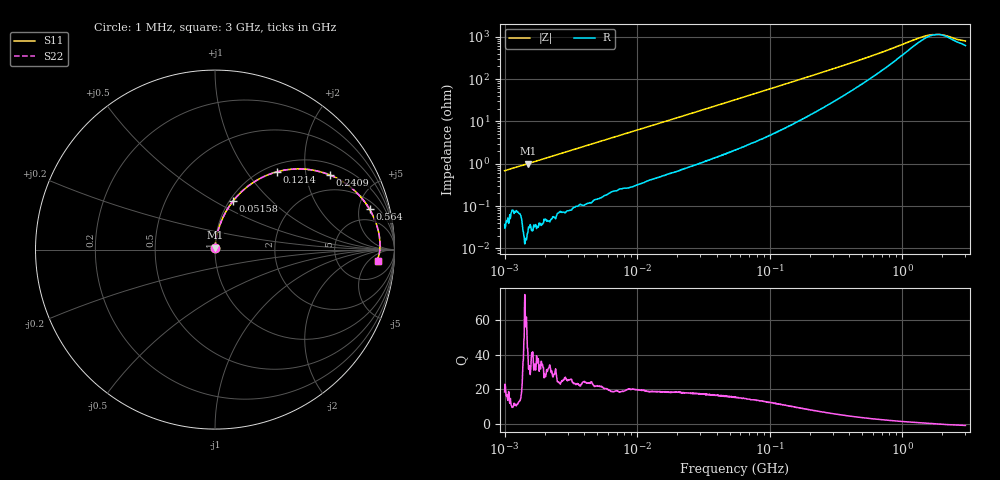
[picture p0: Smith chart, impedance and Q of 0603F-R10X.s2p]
!s-Parameter Generated by FASTRON Sdn. Bhd.
!FASTRON P/N : 0603F-R10X
!Keysight Technologies: E4991B_MY54100416_A.01.15
!Date: Thu Jun 20 13:05:18 2024
!Version  :Rev00  Thu Jun 20 13:05:18 2024
!Data & Calibration Information:
!Freq  S11  S21  S12  S22
!PortZ  Port1:50+j0  Port2:50+j0
!When reading reference impedance value at option line is always used.
! Remarks : This data is being provided solely for informational purposes.
# Hz S dB R 50
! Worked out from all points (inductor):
!   1601 points, 1 MHz to 3 GHz, reference 50 ohm
!   read as one part in series: L = 108 nH near 1.041 MHz
!   highest Q = 41.5 at 1.507 MHz (marker M1), where L = 107 nH
!   self-resonance near 1.883 GHz
!   S11 on the Smith chart (normalised r, x): 1 MHz: 1.00, +0.01; 51.58 MHz: 1.04, +0.61; 121.4 MHz: 1.12, +1.41; 240.9 MHz: 1.38, +2.76; 564 MHz: 2.98, +6.45; 3 GHz: 13, -10
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1000000  -43.30 86.5  -0.00 -0.4  -0.00 -0.4  -43.30 86.5
1507310  -39.90 87.8  -0.00 -0.6  -0.00 -0.6  -39.90 87.8
3804036  -32.20 86.1  -0.01 -1.4  -0.01 -1.4  -32.20 86.1
7977711  -26.00 84.1  -0.03 -2.9  -0.03 -2.9  -26.00 84.1
1.447069e7  -21.10 81.9  -0.08 -5.1  -0.08 -5.1  -21.10 81.9
3.00453e7  -15.10 76.6  -0.23 -10.1  -0.23 -10.1  -15.10 76.6
5.15801e7  -10.80 69.7  -0.54 -16.7  -0.54 -16.7  -10.80 69.7
5.504702e7  -10.30 68.6  -0.60 -17.7  -0.60 -17.7  -10.30 68.6
8.092269e7  -7.59 61.2  -1.12 -24.6  -1.12 -24.6  -7.59 61.2
1.213667e8  -5.12 51.4  -2.11 -33.5  -2.11 -33.5  -5.12 51.4
1.582265e8  -3.82 44.2  -3.08 -39.8  -3.08 -39.8  -3.82 44.2
2.083556e8  -2.77 36.7  -4.40 -46.2  -4.40 -46.2  -2.77 36.7
2.408952e8  -2.33 32.9  -5.23 -49.2  -5.23 -49.2  -2.33 32.9
3.667557e8  -1.47 22.8  -8.07 -55.9  -8.07 -55.9  -1.47 22.8
5.63991e8  -1.01 14.6  -11.60 -58.3  -11.60 -58.3  -1.01 14.6
7.925923e8  -0.83 9.6  -14.70 -55.4  -14.70 -55.4  -0.83 9.6
1.360679e9  -0.73 3.3  -20.20 -32.5  -20.20 -32.5  -0.73 3.3
1.653904e9  -0.73 1.2  -21.60 -13.9  -21.60 -13.9  -0.73 1.2
1.855641e9  -0.74 0.1  -21.80 -1.7  -21.80 -1.7  -0.74 0.1
1.990301e9  -0.74 -0.6  -21.60 6.3  -21.60 6.3  -0.74 -0.6
2.634014e9  -0.84 -3.1  -19.50 27.5  -19.50 27.5  -0.84 -3.1
3e9  -0.84 -4.1  -18.80 34.5  -18.80 34.5  -0.84 -4.1
